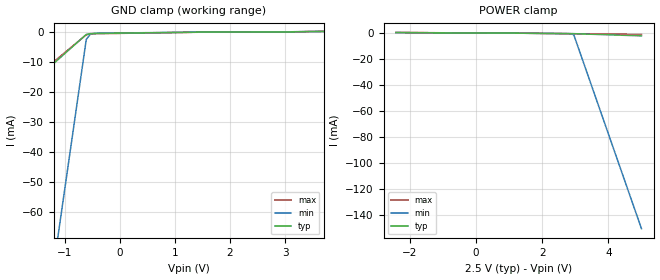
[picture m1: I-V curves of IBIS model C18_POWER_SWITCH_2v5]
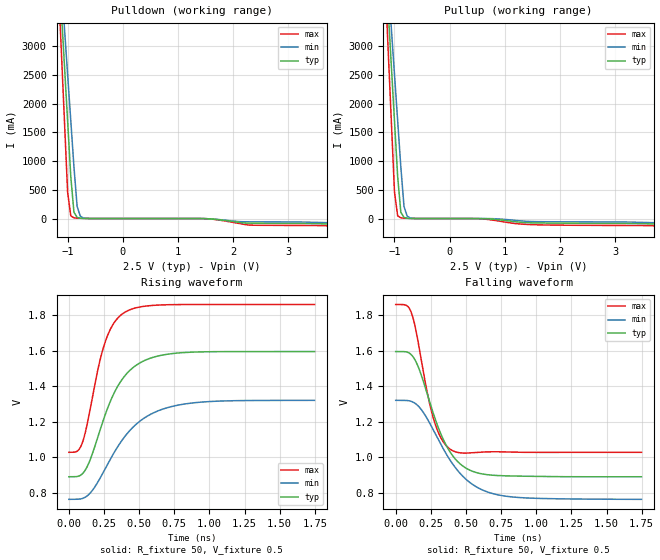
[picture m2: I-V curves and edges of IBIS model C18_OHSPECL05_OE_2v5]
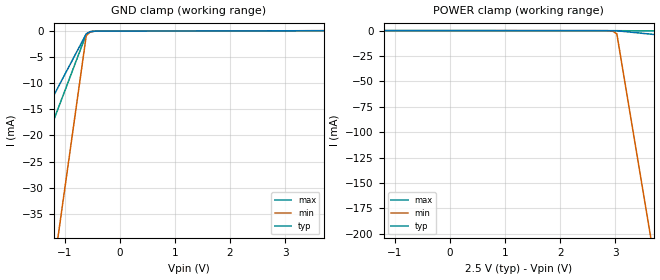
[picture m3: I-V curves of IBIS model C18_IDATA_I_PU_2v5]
|   This file is an IBIS representation of the   |
|   Integrated Device Technology , Inc.   |
|   83PN625I   |
|   PROGRAMMABLE FEMTOCLOCK NG LVPECL OSCILLATOR REPLACEMENT   |
[IBIS Ver]   4.1
[File name]   83pn625i.ibs
[File Rev]   1.0
[Date]   26 Jul 2010
[Source]   Originated at Integrated Device Technology, Inc.
[Disclaimer]
IDT hereby grants the user of this IBIS model a non-exclusive,
nontransferable license to use this IBIS model under the following terms.
Before using this IBIS model, the user should read this license.
If the user does not accept these terms,  the IBIS model should be
returned to IDT within 30 days.
   The user is granted this license only to use the IBIS model and
is not granted rights to sell, load, rent, lease or license the IBIS
model in whole or in part, or in modified form to anyone other than
user. User may modify the IBIS model to suit its specific
applications but rights to derivative works and such modifications
shall belong to IDT.
   This IBIS model is provided on an "AS IS" basis and IDT makes
absolutely no warranty with respect to the information contained
herein. IDT DISCLAIMS AND CUSTOMER WAIVES ALL WARRANTIES, EXPRESS
OR IMPLIED, INCLUDING WARRANTIES OF MERCHANTABILITY OR FITNESS FOR
A PARTICULAR PURPOSE. The entire risk as to quality and performance
is with the Customer. ACCORDINGLY, IN NO EVENT SHALL THE COMPANY BE
LIABLE FOR ANY DAMAGES, WHETHER IN CONTRACT OR TORT,INCLUDING ANY
LOST PROFITS OR OTHER INCIDENTAL, CONSEQUENTIAL, EXEMPLARY, OR
PUNITIVE DAMAGES ARISING OUT OF THE USE OR APPLICATION OF THE IBIS
model provided in this package. Further, IDT reserves the right to
make changes without notice to any product herein to improve
reliability, function, or design. IDT does not convey any license
under patent rights or any other intellectual property rights,
including those of third parties.
   IDT is not obligated to provide maintenance or support
for the licensed IBIS model.
[Copyright]   Copyright 2010 by Integrated Device Technology , Inc.
[Component]   ICS83PN625KI
[Manufacturer] Integrated Device Technology, Inc.
[Package]
|VFQFN 10 Lead
|   typ   min   max
R_pkg   97.2824m   65.7555m   122.0734m
L_pkg   0.3877n   0.3190n   0.4764n
C_pkg   0.0767p   0.0569p   0.0979p
[Pin]   signal_name   model_name   R_pin   L_pin   C_pin
1   OE   C18_POWER_SWITCH   122.0735m   0.3732n   0.0979p
2   RESERVED   NC   71.0181m   0.3190n   0.0784p
3   VEE   GND   107.0351m   0.4274n   0.0964p
4   XTAL_OUT   NC   105.1539m   0.3523n   0.0621p
5   XTAL_IN   NC   109.9892m   0.4744n   0.0628p
6   Q   C18_OHSPECL05_OE   101.2420m   0.3244n   0.0909p
7   nQ   C18_OHSPECL05_OE   65.7555m   0.3335n   0.0733p
8   VCC   POWER   93.3010m   0.4719n   0.0869p
9   FSEL0   C18_IDATA_I_PU   117.5016m   0.3250n   0.0610p
10   FSEL1   C18_INESD01_PU   79.7533m   0.4764n   0.0569p
[Diff Pin]   inv_pin   vdiff   tdelay_typ   tdelay_min   tdelay_max
6   7   NA   0   0   0
[Model Selector] C18_POWER_SWITCH
C18_POWER_SWITCH_2v5  Buffer selection for 2v5
C18_POWER_SWITCH_3v3  Buffer selection for 3v3
[Model Selector] C18_OHSPECL05_OE
C18_OHSPECL05_OE_2v5  Buffer selection for 2v5
C18_OHSPECL05_OE_3v3  Buffer selection for 3v3
[Model Selector] C18_IDATA_I_PU
C18_IDATA_I_PU_2v5  Buffer selection for 2v5
C18_IDATA_I_PU_3v3  Buffer selection for 3v3
[Model Selector] C18_INESD01_PU
C18_INESD01_PU_2v5  Buffer selection for 2v5
C18_INESD01_PU_3v3  Buffer selection for 3v3
| Models and submodels in the file (8): C18_POWER_SWITCH_2v5 (Input), C18_OHSPECL05_OE_2v5 (Output_ECL), C18_IDATA_I_PU_2v5 (Input), C18_INESD01_PU_2v5 (Input), C18_POWER_SWITCH_3v3 (Input), C18_OHSPECL05_OE_3v3 (Output_ECL), C18_IDATA_I_PU_3v3 (Input), C18_INESD01_PU_3v3 (Input)
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[Model] C18_POWER_SWITCH_2v5
Model_type   Input
Polarity   Non-Inverting
Vinl = 0.7V
Vinh = 1.7V
|   typ   min   max
C_comp   2pF   1.5pF   2.5pF
|   typ   min   max
[Voltage range]   2.5V   2.375V   2.625V
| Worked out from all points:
|   GND clamp passes 1 mA (typ) near -0.62 V on its own axis
[GND_clamp]
|Voltage   I (typ)   I (min)   I (max)
-2.424V   -30.6mA    -235mA     -28.61mA
-1.136V   -9.493mA   -70.29mA   -9.004mA
-1.061V   -8.251mA   -60.6mA    -7.851mA
-606.1mV  -801.2uA   -2.477mA   -932.4uA
-530.3mV  -539.6uA   -666.5uA   -636.9uA
-378.8mV  -453.7uA   -388.8uA   -548.2uA
1.364V    -69.12uA   -22.74uA   -85.15uA
5V        417.6uA    364.3uA    500.2uA
[Power_clamp]
|Voltage   I (typ)   I (min)   I (max)
-2.424V   404.7uA    335.7uA    510.7uA
2.727V    -419.4uA   -382uA     -474.1uA
2.879V    -453.7uA   -526uA     -514.5uA
2.955V    -477.4uA   -1.442mA   -534.8uA
5V        -2.158mA   -150.8mA   -1.103mA
[Model] C18_OHSPECL05_OE_2v5
Model_type   Output_ECL
Polarity   Non-Inverting
|   typ   min   max
C_comp   2pF   1.5pF   2.5pF
Vmeas = 1.25V
Rref = 50
Cref = 0
Vref = 0.5V
|   typ   min   max
[Voltage range]   2.5V   2.375V   2.625V
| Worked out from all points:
|   rising waveform, R_fixture 50, V_fixture 0.5: 20-80 % time 222ps typ, 298ps min, 147ps max; typ from 0.89 V to 1.59 V
|   falling waveform, R_fixture 50, V_fixture 0.5: 20-80 % time 200ps typ, 272ps min, 129ps max; typ from 1.59 V to 0.89 V
[Pulldown]
|Voltage   I (typ)   I (min)   I (max)
-2.5V     31.14A     27.8A      36.91A
-1.3V     6.78A      6.74A      6.961A
-1V       1.716A     2.526A     483.4mA
-941.5mV  730.2mA    1.706A     45.91mA
-884.1mV  108.8mA    899.7mA    12.51mA
-826.6mV  20.14mA    210.5mA    6.917mA
-769.2mV  5.982mA    41.46mA    4.556mA
-711.7mV  2.46mA     10.05mA    2.781mA
1.472V    -1.209mA   -1.638mA   -1.061mA
2.276V    -80.57mA   -56.82mA   -112.8mA
3.655V    -92.97mA   -70.89mA   -125.2mA
5V        -139.4mA   -107.3mA   -188.7mA
[Pullup]
|Voltage   I (typ)   I (min)   I (max)
-2.5V     31.14A     27.8A      36.91A
-1.3V     6.78A      6.74A      6.961A
-1V       1.716A     2.526A     483.4mA
-941.5mV  730.2mA    1.706A     45.91mA
-884.1mV  108.8mA    899.7mA    12.51mA
-826.6mV  20.14mA    210.5mA    6.917mA
-769.2mV  5.982mA    41.46mA    4.556mA
-711.7mV  2.46mA     10.05mA    2.781mA
495mV     -87.68uA   -7.314uA   -990.8uA
1.472V    -73.59mA   -51.46mA   -105.4mA
3.598V    -91.45mA   -69.62mA   -123.8mA
5V        -139.3mA   -107.3mA   -188.3mA
[Ramp]
|   typ   min   max
dV/dt_r   0.562/0.353n   0.444/0.472n   0.664/0.232n
dV/dt_f   0.563/0.309n   0.445/0.422n   0.668/0.196n
R_load =   50.0000
[Rising Waveform]
R_fixture = 50
V_fixture = 0.5   | VCC_typ - 2V
V_fixture_max = 0.625   | VCC_max - 2V
V_fixture_min = 0.375   | VCC_min - 2V
C_fixture = 0.0p
| Time   typ   min   max
0s        890.5mV    763.6mV    1.028V
92.84ps   904.4mV    767.5mV    1.074V
150.7ps   983.5mV    797.8mV    1.266V
208.5ps   1.119V     863.1mV    1.499V
255.8ps   1.232V     931mV      1.641V
318.8ps   1.356V     1.022V     1.752V
397.6ps   1.457V     1.116V     1.815V
562.3ps   1.552V     1.233V     1.851V
783ps     1.586V     1.294V     1.858V
1.748ns   1.594V     1.32V      1.859V
[Falling Waveform]
R_fixture = 50
V_fixture = 0.5   | VCC_typ - 2V
V_fixture_max = 0.625   | VCC_max - 2V
V_fixture_min = 0.375   | VCC_min - 2V
C_fixture = 0.0p
| Time   typ   min   max
0s        1.594V     1.32V      1.859V
110.4ps   1.577V     1.314V     1.815V
168.2ps   1.493V     1.281V     1.61V
224.2ps   1.356V     1.217V     1.365V
268ps     1.246V     1.153V     1.22V
325.8ps   1.122V     1.066V     1.103V
395.9ps   1.019V     973.1mV    1.041V
529ps     926.9mV    857.2mV    1.025V
735.7ps   896.9mV    787.5mV    1.031V
1.748ns   890.5mV    763.6mV    1.028V
[Model] C18_IDATA_I_PU_2v5
Model_type   Input
Polarity   Non-Inverting
Vinl = 0.7V
Vinh = 1.7V
|   typ   min   max
C_comp   2pF   1.5pF   2.5pF
|   typ   min   max
[Voltage range]   2.5V   2.375V   2.625V
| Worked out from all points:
|   GND clamp passes 1 mA (typ) near -0.63 V on its own axis
[GND_clamp]
|Voltage   I (typ)   I (min)   I (max)
-2.5V     -38.44mA   -143.2mA   -53.29mA
-2.424V   -36.93mA   -137.5mA   -51.19mA
-1.97V    -27.84mA   -103.3mA   -38.56mA
-1.894V   -26.32mA   -97.64mA   -36.45mA
-1.136V   -11.17mA   -40.73mA   -15.4mA
-1.061V   -9.653mA   -35.04mA   -13.29mA
-606.1mV  -561.9uA   -894.9uA   -660.6uA
-530.3mV  -155.5uA   -183.2uA   -155.3uA
-303mV    -56.19uA   -50.54uA   -62.19uA
5V        49.97uA    49.09uA    50.42uA
[Power_clamp]
|Voltage   I (typ)   I (min)   I (max)
-2.5V     49.97uA    46.75uA    53.08uA
2.955V    -73.26uA   -484.1uA   -62.81uA
3.03V     -155.5uA   -3.162mA   -65.88uA
3.561V    -3.001mA   -176mA     -211.6uA
3.636V    -3.407mA   -200.7mA   -232.4uA
5V        -10.72mA   -645.2mA   -607uA
